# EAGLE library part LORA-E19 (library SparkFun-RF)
Chengdu Ebyte E19-915M30S - 915/868/433MHz LoRa (FSK) TRX Using SX1276 This is a LoRa (or optionally FSK) modulated transciver bassed on the Semtech SX1276. It has a high ouput power of 1W an a pre-installed U.FL connector. Can be used with LoRa WAN with DIO0, DIO1, and DIO2 hooked up to controller interrupt inputs SparkFun Products: SAMD21 Pro RF 1W
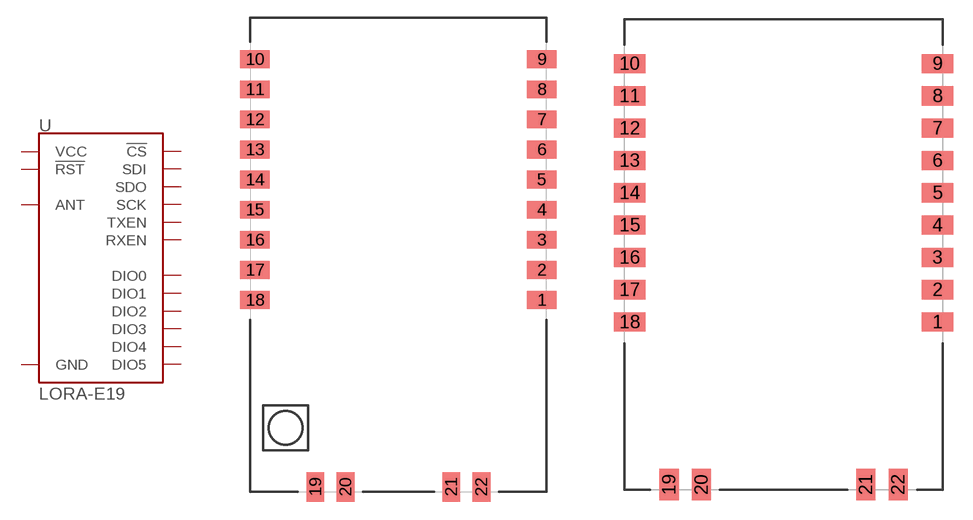
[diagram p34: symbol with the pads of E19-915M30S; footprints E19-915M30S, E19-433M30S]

Designator prefix U

## LORA-E19915MHZ (PROD_ID: IC-14076)  [E19-915M30S]
1  GND
2  DIO5
3  DIO4
4  DIO3
5  DIO2
6  DIO1
7  DIO0
8  !RST
9  GND
10  GND
11  VCC
12  SCK
13  SDO
14  SDI
15  !CS
16  TXEN
17  RXEN
18  GND
19  ANT
20  GND
21  GND
22  GND

## LORA-E19868MHZ (PROD_ID: IC-16573)  [E19-915M30S]
Pads as for E19-915M30S

## LORA-E19433MHZ (PROD_ID: IC-16574)  [E19-433M30S]
Pads as for E19-915M30S

## Footprint E19-915M30S (pad centres in mm)
E19-915M30S - 1W 915MHz TRX Using SX1276 Specifications: Pin count: 22 Pin pitch: Varies Area: 1.15 in x 1.65 in Datasheet referenced for footprint Example device(s): SAMD21 ProRF 1W
smd 2.5 x 1.5: 1 12.1,-3.82; 2 12.1,-1.28; 3 12.1,1.26; 4 12.1,3.8; 5 12.1,6.34; 6 12.1,8.88; 7 12.1,11.42; 8 12.1,13.96; 9 12.1,16.5; 10 -12.1,16.5; 11 -12.1,13.96; 12 -12.1,11.42; 13 -12.1,8.88; 14 -12.1,6.34; 15 -12.1,3.8; 16 -12.1,1.26; 17 -12.1,-1.28; 18 -12.1,-3.82
smd 1.5 x 2.5: 19 -7,-19.6; 20 -4.46,-19.6; 21 4.46,-19.6; 22 7,-19.6

## Footprint E19-433M30S (pad centres in mm)
E19-915M30S - 1W 433MHz TRX Using SX1276
smd 2.5 x 1.5: 1 12.1,-5.32; 2 12.1,-2.78; 3 12.1,-0.24; 4 12.1,2.3; 5 12.1,4.84; 6 12.1,7.38; 7 12.1,9.92; 8 12.1,12.46; 9 12.1,15; 10 -12.1,15; 11 -12.1,12.46; 12 -12.1,9.92; 13 -12.1,7.38; 14 -12.1,4.84; 15 -12.1,2.3; 16 -12.1,-0.24; 17 -12.1,-2.78; 18 -12.1,-5.32
smd 1.5 x 2.5: 19 -9,-18.1; 20 -6.46,-18.1; 21 6.46,-18.1; 22 9,-18.1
